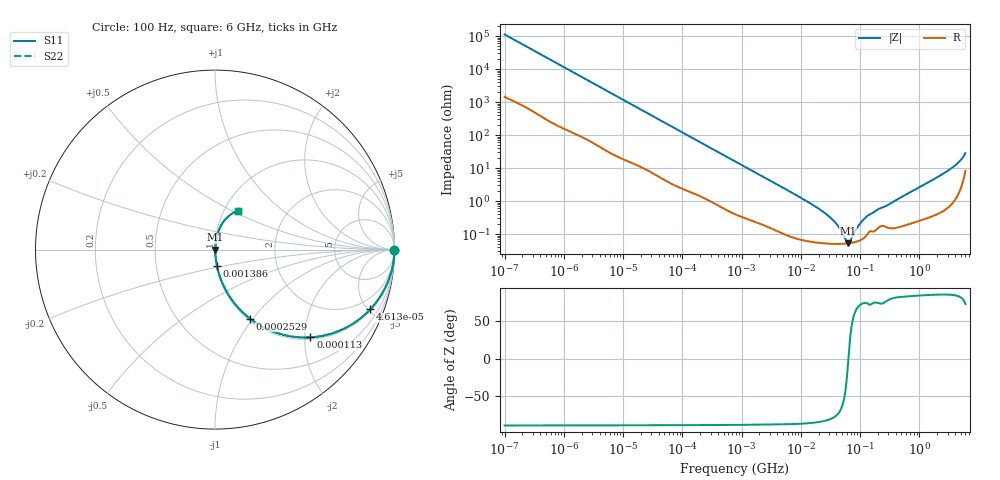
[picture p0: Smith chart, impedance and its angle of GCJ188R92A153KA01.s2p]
!Murata Part Number: GCJ188R92A153KA01
!These Parameters are Measured in Series Mode Connection
!Data Generated on Mar 13, 2026
!  o--ll--o
!Port1  Port2
!  o------o
!Operation Temp=25[degC], DC Bias Voltage=0[V]
!Freq. Start=100[Hz] Stop=6[GHz] 401[Steps]
# Hz S RI R 50
!Freq.(Hz) S11(Real) S11(Imag) S21(Real) S21(Imag) S12(Real) S12(Imag) S22(Real) S22(Imag)
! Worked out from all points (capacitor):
!   401 points, 100 Hz to 6 GHz, reference 50 ohm
!   read as one part in series: C = 14.1 nF near 109 Hz
!   lowest |Z| = 52.9 mohm at 62.33 MHz (marker M1)
!   series resonance near 63.55 MHz, so ESL is about 440 pH
!   S11 on the Smith chart (normalised r, x): 100 Hz: open; 46.13 kHz: 1.09, -5.18; 113 kHz: 1.04, -2.13; 252.9 kHz: 1.02, -0.96; 1.386 MHz: 1.01, -0.18; 6 GHz: 1.17, +0.54
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100  1 -0.000888  1.22e-05 0.000888  1.22e-05 0.000888  1 -0.000888
2008  0.9994 -0.0174  0.000568 0.0174  0.000568 0.0174  0.9994 -0.0174
11514  0.9889 -0.0968  0.0111 0.0968  0.0111 0.0968  0.9889 -0.0968
40335  0.893 -0.3  0.107 0.3  0.107 0.3  0.893 -0.3
46134  0.8657 -0.3319  0.1343 0.3319  0.1343 0.3319  0.8657 -0.3319
112960  0.5317 -0.489  0.4683 0.489  0.4683 0.489  0.5317 -0.489
252896  0.1945 -0.3841  0.8055 0.3841  0.8055 0.3841  0.1945 -0.3841
413847  0.0865 -0.2694  0.9135 0.2694  0.9135 0.2694  0.0865 -0.2694
774597  0.0286 -0.1547  0.9714 0.1547  0.9714 0.1547  0.0286 -0.1547
1386327  0.0107 -0.0889  0.9893 0.0889  0.9893 0.0889  0.0107 -0.0889
1.555665e7  0.000638 -0.00783  0.9994 0.00783  0.9994 0.00783  0.000638 -0.00783
3.64232e7  0.000509 -0.00241  0.9995 0.00241  0.9995 0.00241  0.000509 -0.00241
4.556224e7  0.000505 -0.0014  0.9995 0.0014  0.9995 0.0014  0.000505 -0.0014
5.699437e7  0.000515 -0.000451  0.9995 0.000451  0.9995 0.000451  0.000515 -0.000451
6.233367e7  0.000523 -7.94e-05  0.9995 7.94e-05  0.9995 7.94e-05  0.000523 -7.94e-05
6.817316e7  0.000535 0.000292  0.9995 -0.000292  0.9995 -0.000292  0.000535 0.000292
9.326766e7  0.000616 0.00164  0.9994 -0.00164  0.9994 -0.00164  0.000616 0.00164
1.275994e8  0.000903 0.0032  0.9991 -0.0032  0.9991 -0.0032  0.000903 0.0032
3.124326e8  0.00157 0.00792  0.9984 -0.00792  0.9984 -0.00792  0.00157 0.00792
2.802721e9  0.0112 0.0745  0.9888 -0.0745  0.9888 -0.0745  0.0112 0.0745
4.193612e9  0.0275 0.1223  0.9725 -0.1223  0.9725 -0.1223  0.0275 0.1223
6e9  0.1309 0.2176  0.8691 -0.2176  0.8691 -0.2176  0.1309 0.2176
